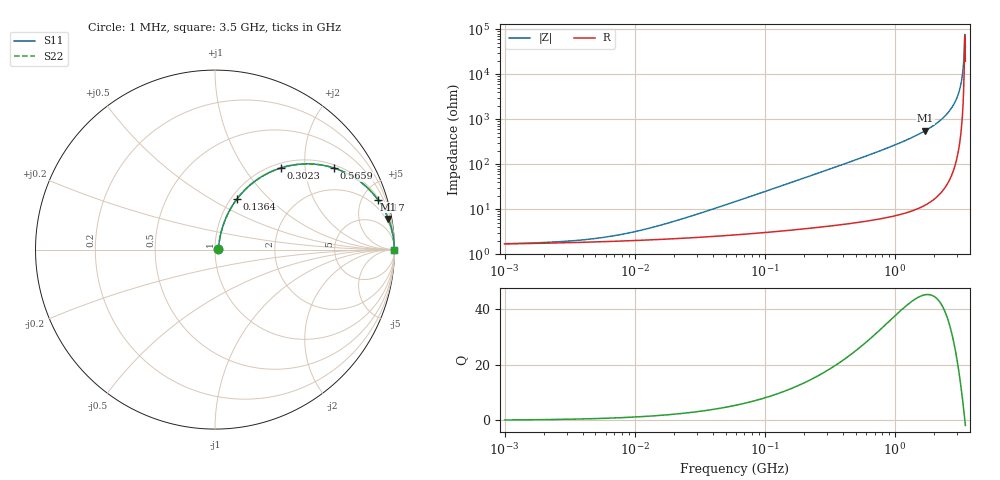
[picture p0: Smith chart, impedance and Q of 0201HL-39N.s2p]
# MHz  S  MA  R  50
!Freq  MagS11  AngS11  MagS21  AngS21  MagS12  AngS12  MagS22  AngS22
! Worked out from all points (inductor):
!   822 points, 1 MHz to 3.5 GHz, reference 50 ohm
!   read as one part in series: L = 39 nH near 28.88 MHz
!   highest Q = 45.1 at 1.725 GHz (marker M1), where L = 51.8 nH
!   self-resonance near 3.461 GHz
!   S11 on the Smith chart (normalised r, x): 1 MHz: 1.03, +0.00; 136.4 MHz: 1.07, +0.67; 302.3 MHz: 1.08, +1.49; 565.9 MHz: 1.11, +2.85; 1.17 GHz: 1.16, +6.47; 3.5 GHz: open
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1  0.01687 8.1  0.9833 -0.1  0.9833 -0.1  0.01687 8.1
3.908663  0.0204 26.9  0.9819 -0.5  0.9819 -0.5  0.0204 26.9
7.689208  0.02667 42.8  0.9806 -1.1  0.9806 -1.1  0.02667 42.8
15.27765  0.04215 58.3  0.9785 -2.1  0.9785 -2.1  0.04215 58.3
59.71516  0.1435 71.4  0.964 -8.1  0.964 -8.1  0.1435 71.4
136.3825  0.3098 66.4  0.921 -18.0  0.921 -18.0  0.3098 66.4
231.0955  0.4815 57.4  0.8447 -28.7  0.8447 -28.7  0.4815 57.4
302.3212  0.5834 51.2  0.7803 -35.6  0.7803 -35.6  0.5834 51.2
565.868  0.8048 34.3  0.5645 -53.5  0.5645 -53.5  0.8048 34.3
903.2743  0.9125 22.6  0.3842 -65.8  0.3842 -65.8  0.9125 22.6
1169.972  0.9488 17.0  0.2932 -71.5  0.2932 -71.5  0.9488 17.0
1724.682  0.9808 10.1  0.1746 -78.7  0.1746 -78.7  0.9808 10.1
2395.048  0.9939 5.1  0.08857 -83.5  0.08857 -83.5  0.9939 5.1
2672.08  0.9962 3.5  0.06183 -84.7  0.06183 -84.7  0.9962 3.5
2922.414  0.9976 2.3  0.0404 -85.4  0.0404 -85.4  0.9976 2.3
3102.202  0.9982 1.5  0.02627 -85.4  0.02627 -85.4  0.9982 1.5
3228.163  0.9985 1.0  0.0169 -84.4  0.0169 -84.4  0.9985 1.0
3293.05  0.9986 0.7  0.01223 -83.2  0.01223 -83.2  0.9986 0.7
3325.98  0.9987 0.6  0.009907 -82.0  0.009907 -82.0  0.9987 0.6
3392.832  0.9987 0.3  0.005294 -76.0  0.005294 -76.0  0.9987 0.3
3495.638  0.9988 -0.1  0.002221 57.3  0.002221 57.3  0.9988 -0.1
3500  0.9988 -0.1  0.002472 61.0  0.002472 61.0  0.9988 -0.1
